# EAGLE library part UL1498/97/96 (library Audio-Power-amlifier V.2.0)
AF AMPLIEFIERS 1,2W
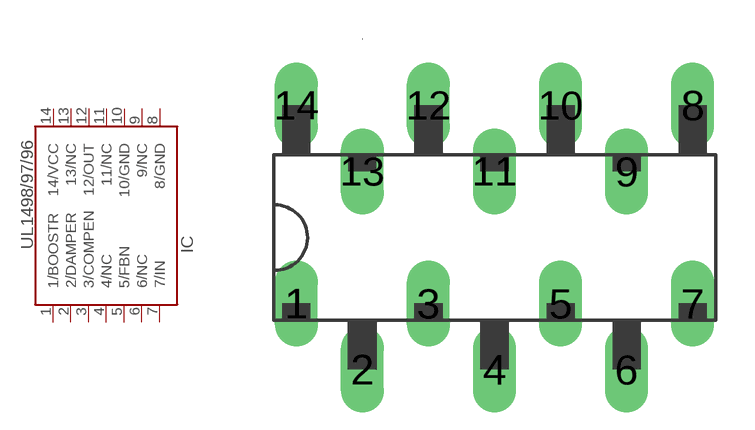
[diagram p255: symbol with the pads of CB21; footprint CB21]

Designator prefix IC

## UL1498/97/96  [CB21]
1  1/BOOSTR
2  2/DAMPER
3  3/COMPEN
4  4/NC  nc
5  5/FBN
6  6/NC  nc
7  7/IN  in
8  8/GND  pwr
9  9/NC  nc
10  10/GND  pwr
11  11/NC  nc
12  12/OUT  out
13  13/NC  nc
14  14/VCC  pwr

## Footprint CB21 (pad centres in mm)
drill 1.1 long: 1 -7.62,-2.54; 2 -5.08,-5.08; 3 -2.54,-2.54; 4 0,-5.08; 5 2.54,-2.54; 6 5.08,-5.08; 7 7.62,-2.54; 8 7.62,5.08; 9 5.08,2.54; 10 2.54,5.08; 11 0,2.54; 12 -2.54,5.08; 13 -5.08,2.54; 14 -7.62,5.08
